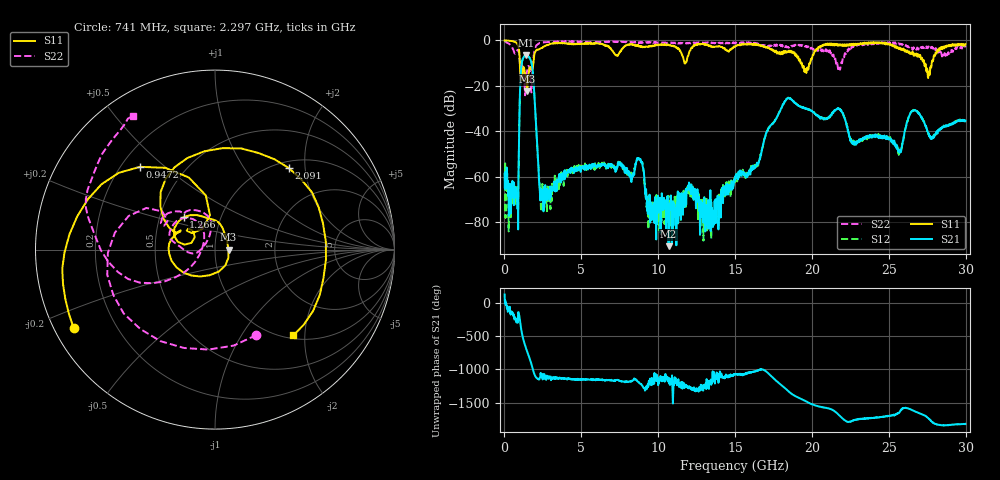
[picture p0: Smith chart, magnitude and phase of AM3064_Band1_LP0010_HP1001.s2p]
# Hz S DB R 50.0
!freq dBS11 angS11 dBS21 angS21 dBS12 angS12 dBS22 angS22
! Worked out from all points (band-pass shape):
!   1600 points, 10 MHz to 29.98 GHz, reference 50 ohm
!   highest |S21| = -6.40 dB at 1.397 GHz (marker M1); lowest = -90.6 dB at 10.68 GHz (marker M2)
!   |S21| within 3 dB of the highest: 1.143 GHz to 1.738 GHz (595.4 MHz wide, 41.3 % of centre)
!   lowest |S11| = -22.4 dB at 1.472 GHz (marker M3), VSWR 1.16, Z = 58.2 - j0.0264 ohm
!   |S11| at or under -10 dB: 1.002 GHz to 1.878 GHz (876.3 MHz wide, 60.9 % of centre); 19.34 GHz to 19.89 GHz (544.4 MHz wide, 2.78 % of centre); 27.3 GHz to 27.8 GHz (497.1 MHz wide, 1.8 % of centre)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
!   |S22| runs from -24.2 to -0.3 dB; largest |S21 - S12| = 0.0053
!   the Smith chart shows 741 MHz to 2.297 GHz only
!   S11 on the Smith chart (normalised r, x): 741 MHz: 0.06, -0.26; 947.2 MHz: 0.28, +0.42; 1.266 GHz: 0.66, +0.26; 2.091 GHz: 1.13, +1.64; 2.297 GHz: 1.06, -1.75
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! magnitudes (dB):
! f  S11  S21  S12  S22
! 10 MHz  0.0  -59.0  -59.1  -0.3
! 741 MHz  -0.9  -68.0  -67.4  -5.5
! 947.2 MHz  -4.1  -44.3  -44.0  -5.7
! 1.116 GHz  -15.9  -10.5  -10.4  -10.8
! 1.266 GHz  -12.0  -7.2  -7.2  -14.3
! 1.397 GHz  -16.5  -6.4  -6.4  -17.9
! 1.472 GHz  -22.4  -6.5  -6.5  -13.3
! 1.809 GHz  -13.2  -11.8  -11.7  -15.3
! 2.091 GHz  -4.3  -41.4  -41.4  -2.1
! 2.297 GHz  -3.8  -65.9  -63.5  -1.2
! 5.015 GHz  -1.5  -55.7  -56.6  -0.6
! 8.782 GHz  -2.7  -52.6  -52.3  -0.9
! 10 GHz  -2.0  -75.8  -74.9  -0.9
! 10.68 GHz  -1.9  -90.6  -68.5  -1.0
! 13.52 GHz  -3.0  -79.3  -75.4  -1.2
! 15 GHz  -2.8  -59.9  -61.6  -1.3
! 18.34 GHz  -5.5  -25.8  -25.8  -2.6
! 19.99 GHz  -8.2  -31.2  -31.2  -3.4
! 25 GHz  -1.4  -43.7  -43.4  -1.1
! 26.64 GHz  -6.5  -30.8  -30.8  -3.5
! 27.56 GHz  -16.5  -40.7  -41.4  -2.8
! 29.98 GHz  -1.6  -35.3  -35.9  -3.1
